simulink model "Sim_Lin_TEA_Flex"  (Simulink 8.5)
settings: Solver=ode23  StartTime=0.0  StopTime=108000  RelTol=1e-3
InitFcn:
  | start
StopFcn:
  | pl2
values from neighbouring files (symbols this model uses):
  Kpqr = lqr(sys,Q0,R0)    [des.m]
  wo = 0.0011    [start.m]    (also in start1.m; start2.m; start3.m)
undefined symbols (not defined in the file or in its folder): Af, Bf, Cf, Df

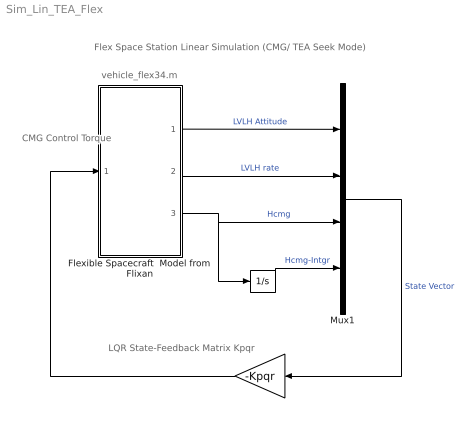
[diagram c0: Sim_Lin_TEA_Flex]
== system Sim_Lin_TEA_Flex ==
  note: Flex Space Station Linear Simulation (CMG/ TEA Seek Mode)
  note: LQR State-Feedback Matrix Kpqr
  note: CMG Control Torque
  note: vehicle_flex34.m
  " " : Gain  Gain=-Kpqr  Multiplication=Matrix(K*u)
  "  " : Integrator
  Flexible Spacecraft  Model from Flixan : Subsystem
  Mux1 : Mux  Inputs=[3, 3, 3, 3]
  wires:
  "  "/1 -> Mux1/4  "Hcmg-Intgr"
  " "/1 -> Flexible Spacecraft  Model from Flixan/1(Tcmg)
  Mux1/1 -> " "/1  "State Vector"
  Flexible Spacecraft  Model from Flixan/3("Hcmg ") -> Mux1/3, "  "/1  "Hcmg"
  Flexible Spacecraft  Model from Flixan/2(w-lv) -> Mux1/2  "LVLH rate"
  Flexible Spacecraft  Model from Flixan/1(att-lv) -> Mux1/1  "LVLH Attitude"

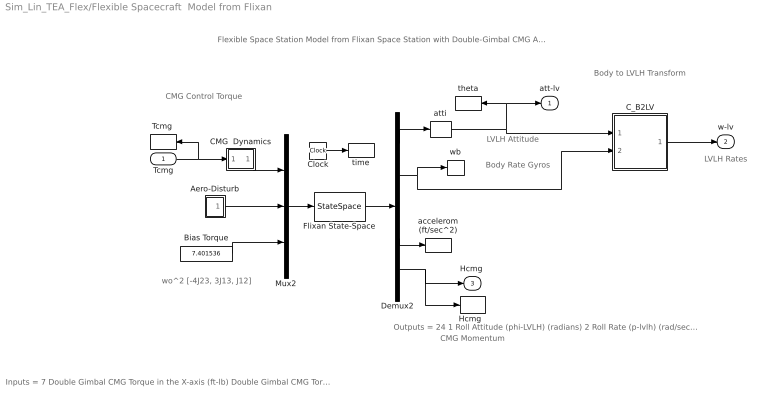
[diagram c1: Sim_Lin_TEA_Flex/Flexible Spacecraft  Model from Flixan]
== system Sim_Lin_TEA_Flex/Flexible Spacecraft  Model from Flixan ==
  note: Body to LVLH Transform
  note: wo^2 [-4J23, 3J13, J12]
  note: CMG Momentum
  note: LVLH Attitude
  note: LVLH Rates
  note: Body Rate Gyros
  note: CMG Control Torque
  note: Outputs = 24 1 Roll Attitude (phi-LVLH) (radians) 2 Roll Rate (p-lvlh) (rad/sec) 3 Pitch Attitude (thet-LVLH) (radians) 4 Pitch Rate (q-lvlh) (rad/sec) 5 Yaw Attitude (psi-LVLH) (radians) 6 Yaw Rate (r-lvlh) (rad/sec) 7 Angle of attack, alfa, (radians) 8 Angle of sideslip, beta, (radian) 9 Change in Altitude, delta-h, (feet) 10 Forward Acceleration (V-dot) (ft/sec) 11 Cross Range Velocity (Vcr) (ft/sec) 12 Rate-Gyro # 1, Roll Rate (Body) (rad/sec) 13 Rate-Gyro # 2, Pitch Rate (Body) (rad/sec) 14 Rate-Gyro # 3, Yaw Rate (Body) (rad/sec) 15 Gyro # 4, Roll Attitude (Body) (radians) 16 Gyro # 5, Pitch Attitude (Body) (radians) 17 Gyro # 6, Yaw Attitude (Body) (radians) 18 Accelerom # 1, (along X), (ft/sec^2) Translat. Accelerat. 19 Accelerom # 2, (along Z), (ft/sec^2) Translat. Accelerat. 20 Accelerom # 3, (along X), (ft/sec^2) Translat. Accelerat. 21 Accelerom # 4, (along Z), (ft/sec^2) Translat. Accelerat. 22 Double Gimbal CMG Momentum Change in X-axis (ft-lb-sec) 23 Double Gimbal CMG Momentum Change in Y-axis (ft-lb-sec) 24 Double Gimbal CMG Momentum Change in Z-axis (ft-lb-sec)
  note: Inputs = 7 Double Gimbal CMG Torque in the X-axis (ft-lb) Double Gimbal CMG Torque in the Y-axis (ft-lb) Double Gimbal CMG Torque in the Z-axis (ft-lb) External Torque Input 1 (ft-lb), direct: External Torque Input 2 (ft-lb), direct: External Torque Input 3 (ft-lb), direct: Ext Torque Direct.=(0.197, -0.5964, -0.7782)
  note: Flexible Space Station Model from Flixan Space Station with Double-Gimbal CMG Array (Flex)
  Tcmg : Inport  PortDimensions=3
  Aero-Disturb : Subsystem
  Bias Torque : Constant  Value=7.401536
  CMG  Dynamics : Subsystem
  C_B2LV : Subsystem
  Clock : Clock
  Demux2 : Demux  Outputs=[11, 3, 3, 4, 3]
  Flixan State-Space : StateSpace  A=Af  B=Bf  C=Cf  D=Df  X0=0
  "Hcmg  " : ToWorkspace  VariableName=Hcmg  SampleTime=-1
  Mux2 : Mux  Inputs=[3, 3, 1]
  "Tcmg " : ToWorkspace  VariableName=Tcmg  SampleTime=-1
  accelerom (ft/sec^2) : ToWorkspace  VariableName=accel  SampleTime=-1
  atti : Selector  InputPortWidth=11  Indices=[1 3 5]
  theta : ToWorkspace  VariableName=theta  SampleTime=-1
  time : ToWorkspace  VariableName=time  SampleTime=-1
  wb : ToWorkspace  VariableName=wb  SampleTime=-1
  att-lv : Outport
  w-lv : Outport  Port=2
  "Hcmg " : Outport  Port=3
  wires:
  CMG  Dynamics/1(O) -> Mux2/1
  C_B2LV/1(wlv) -> w-lv/1
  Mux2/1 -> Flixan State-Space/1
  Flixan State-Space/1 -> Demux2/1
  Bias Torque/1 -> Mux2/3
  Clock/1 -> time/1
  Demux2/5 -> "Hcmg  "/1, "Hcmg "/1
  Demux2/1 -> atti/1
  atti/1 -> theta/1, att-lv/1, C_B2LV/1(atti)
  Demux2/4 -> accelerom (ft/sec^2)/1
  Demux2/2 -> wb/1, C_B2LV/2(wb)
  Tcmg/1 -> "Tcmg "/1, CMG  Dynamics/1(I)
  Aero-Disturb/1(Td) -> Mux2/2

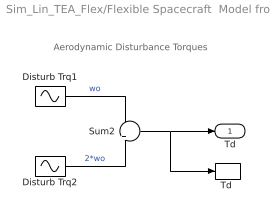
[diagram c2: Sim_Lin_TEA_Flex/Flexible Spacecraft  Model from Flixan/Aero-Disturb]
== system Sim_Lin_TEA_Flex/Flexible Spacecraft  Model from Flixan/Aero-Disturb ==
  note: Aerodynamic Disturbance Torques
  Disturb Trq1 : Sin  Amplitude=[1, 3, 1]  Bias="[1  8  1]"  Frequency=[wo, wo, wo]  SampleTime=0
  Disturb Trq2 : Sin  Amplitude=[1, 1, 1]*0.5  Frequency=[wo, wo, wo]*2  SampleTime=0
  Sum2 : Sum  Inputs=+|+
  "Td " : ToWorkspace  VariableName=Td  SampleTime=-1
  Td : Outport
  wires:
  Disturb Trq1/1 -> Sum2/1  "wo"
  Sum2/1 -> Td/1, "Td "/1
  Disturb Trq2/1 -> Sum2/2  "2*wo"

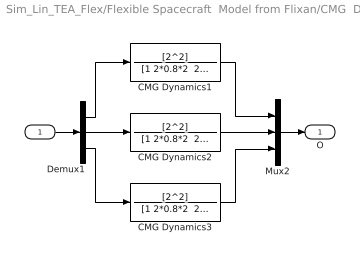
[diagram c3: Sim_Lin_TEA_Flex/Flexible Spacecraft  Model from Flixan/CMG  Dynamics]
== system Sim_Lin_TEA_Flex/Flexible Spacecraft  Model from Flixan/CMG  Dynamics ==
  I : Inport
  CMG Dynamics1 : TransferFcn  Numerator=[2^2]  Denominator="[1 2*0.8*2  2^2]"
  CMG Dynamics2 : TransferFcn  Numerator=[2^2]  Denominator="[1 2*0.8*2  2^2]"
  CMG Dynamics3 : TransferFcn  Numerator=[2^2]  Denominator="[1 2*0.8*2  2^2]"
  Demux1 : Demux  Outputs=3
  Mux2 : Mux  Inputs=3
  O : Outport
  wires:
  CMG Dynamics2/1 -> Mux2/2
  CMG Dynamics3/1 -> Mux2/3
  CMG Dynamics1/1 -> Mux2/1
  Demux1/2 -> CMG Dynamics2/1
  Demux1/1 -> CMG Dynamics1/1
  Demux1/3 -> CMG Dynamics3/1
  I/1 -> Demux1/1
  Mux2/1 -> O/1

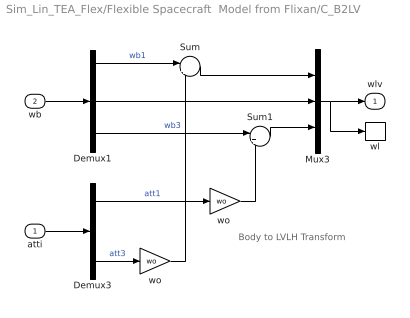
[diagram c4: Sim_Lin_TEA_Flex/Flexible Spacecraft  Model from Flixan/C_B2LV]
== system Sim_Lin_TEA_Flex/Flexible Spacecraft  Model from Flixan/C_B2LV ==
  note: Body to LVLH Transform
  atti : Inport  PortDimensions=3
  wb : Inport  Port=2  PortDimensions=3
  Demux1 : Demux  Outputs=3
  Demux3 : Demux  Outputs=3
  Mux3 : Mux  Inputs=3
  Sum : Sum  Inputs=|++
  Sum1 : Sum  Inputs=|+-
  wl : ToWorkspace  VariableName=wl  SampleTime=-1
  wo : Gain  Gain=wo
  "wo " : Gain  Gain=wo
  wlv : Outport
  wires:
  Demux1/1 -> Sum/1  "wb1"
  Sum/1 -> Mux3/1
  Demux3/3 -> wo/1  "att3"
  Sum1/1 -> Mux3/3
  atti/1 -> Demux3/1
  wb/1 -> Demux1/1
  Mux3/1 -> wlv/1, wl/1
  Demux3/1 -> "wo "/1  "att1"
  Demux1/2 -> Mux3/2
  wo/1 -> Sum/2
  Demux1/3 -> Sum1/1  "wb3"
  "wo "/1 -> Sum1/2
